FUNCTION "FC_PROG_L2" : VOID
TITLE =FC PROG OVEN LINE 2
{ S7_language := '9(1) Angielski (Stany Zjednoczone)  11.01.2022  09:45:15' }
VERSION : 0.1


VAR_TEMP
  DoorOK : BOOL ;
  ECooling_SP : REAL ;
END_VAR
BEGIN
NETWORK
TITLE =SET FULL PRODUCTION OR REDUCED PRODUCTION MODE
//THIS MODE WILL BE USE AFTER IN SETTING SETPOINTS FOR OVEN FANS (=55FAN01,
//=60FAN01)
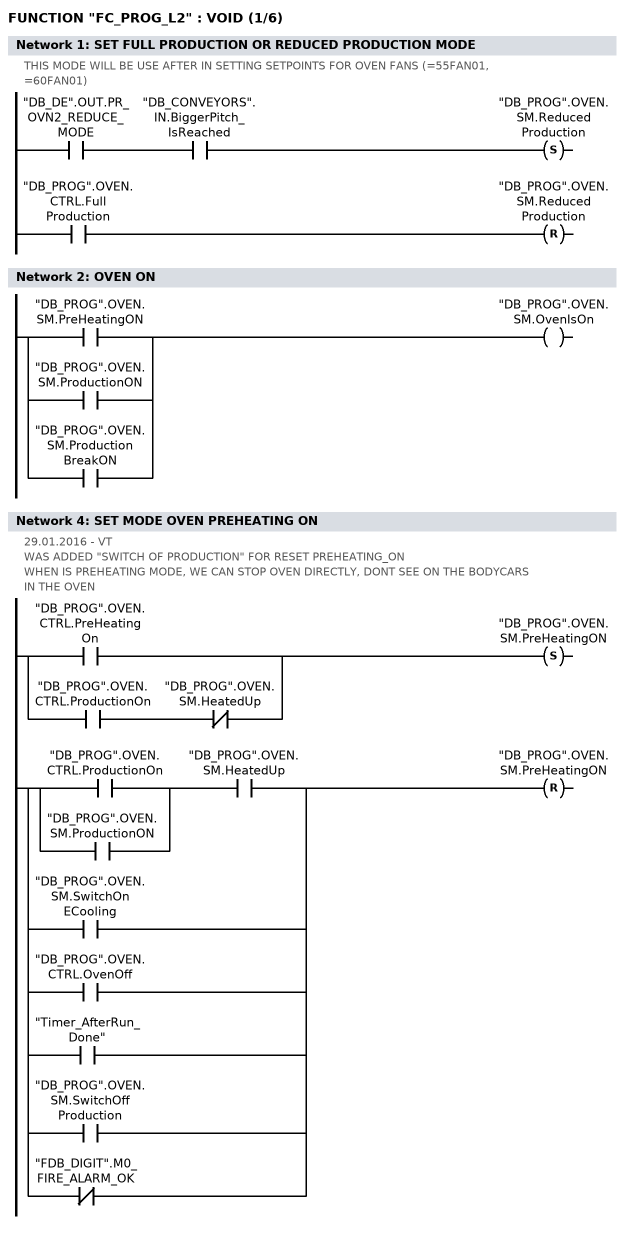
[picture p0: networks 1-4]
      U     "DB_DE".OUT.PR_OVN2_REDUCE_MODE;
      U     "DB_CONVEYORS".IN.BiggerPitch_IsReached;
      S     "DB_PROG".OVEN.SM.ReducedProduction;
      U     "DB_PROG".OVEN.CTRL.FullProduction;
      R     "DB_PROG".OVEN.SM.ReducedProduction;
      NOP   0;
NETWORK
TITLE =OVEN ON

      O     "DB_PROG".OVEN.SM.PreHeatingON;
      O     "DB_PROG".OVEN.SM.ProductionON;
      O     "DB_PROG".OVEN.SM.ProductionBreakON;
      =     "DB_PROG".OVEN.SM.OvenIsOn;
NETWORK
TITLE =SET MODE OF OVEN
//
//************************** SET MODE OF OVEN **********************************
//
NETWORK
TITLE =SET MODE OVEN PREHEATING ON
//29.01.2016 - VT
//WAS ADDED "SWITCH OF PRODUCTION" FOR RESET PREHEATING_ON
//WHEN IS PREHEATING MODE, WE CAN STOP OVEN DIRECTLY, DONT SEE ON THE BODYCARS
//IN THE OVEN
//
//
      U(    ;
      O     "DB_PROG".OVEN.CTRL.PreHeatingOn;
      O     ;
      U     "DB_PROG".OVEN.CTRL.ProductionOn;
      UN    "DB_PROG".OVEN.SM.HeatedUp;
      )     ;
      S     "DB_PROG".OVEN.SM.PreHeatingON;
      U(    ;
      U(    ;
      O     "DB_PROG".OVEN.CTRL.ProductionOn;
      O     "DB_PROG".OVEN.SM.ProductionON;
      )     ;
      U     "DB_PROG".OVEN.SM.HeatedUp;
      O     "DB_PROG".OVEN.SM.SwitchOnECooling;
      O     "DB_PROG".OVEN.CTRL.OvenOff;
      O     "Timer_AfterRun_Done";
      O     "DB_PROG".OVEN.SM.SwitchOffProduction;
      ON    "FDB_DIGIT".M0_FIRE_ALARM_OK;
      )     ;
      R     "DB_PROG".OVEN.SM.PreHeatingON;
      NOP   0;
NETWORK
TITLE =SET MODE OVEN PRODUCTION ON
//29.01.2016 - VT
//WAS ADDED ADDITIONAL LOCK FOR RESER PRODUCTION MODE -
//"OVEN_OFF_AFTER_RUN" (M410.0)
//IT MEANS, THAT WE CAN'T STOP OVEN, WHEN WITH BODYCARS INSIDE
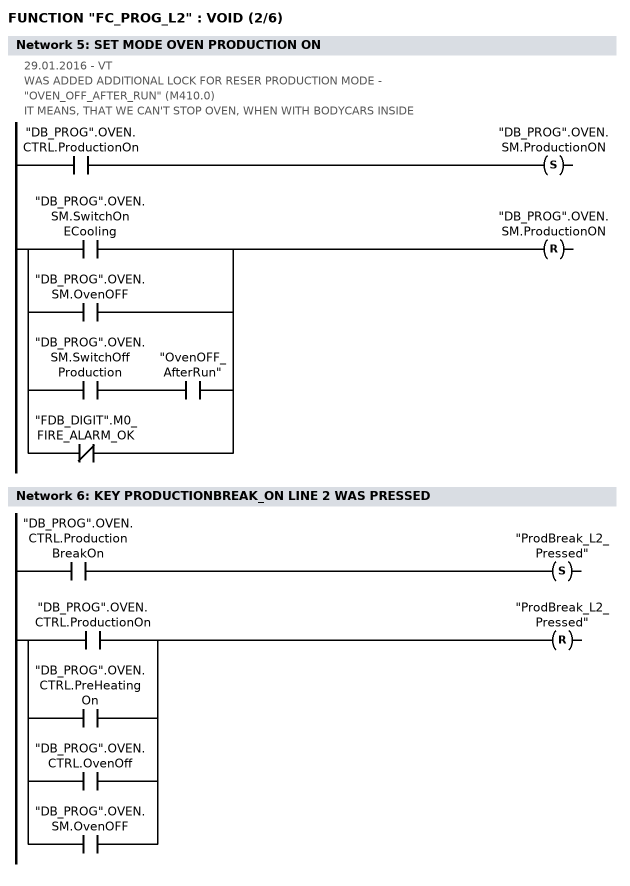
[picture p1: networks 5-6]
      U     "DB_PROG".OVEN.CTRL.ProductionOn;
      S     "DB_PROG".OVEN.SM.ProductionON;
      U(    ;
      O     "DB_PROG".OVEN.SM.SwitchOnECooling;
      O     "DB_PROG".OVEN.SM.OvenOFF;
      O     ;
      U     "DB_PROG".OVEN.SM.SwitchOffProduction;
      U     "OvenOFF_AfterRun";
      ON    "FDB_DIGIT".M0_FIRE_ALARM_OK;
      )     ;
      R     "DB_PROG".OVEN.SM.ProductionON;
      NOP   0;
NETWORK
TITLE =KEY PRODUCTIONBREAK_ON LINE 2 WAS PRESSED

      U     "DB_PROG".OVEN.CTRL.ProductionBreakOn;
      S     "ProdBreak_L2_Pressed";
      U(    ;
      O     "DB_PROG".OVEN.CTRL.ProductionOn;
      O     "DB_PROG".OVEN.CTRL.PreHeatingOn;
      O     "DB_PROG".OVEN.CTRL.OvenOff;
      O     "DB_PROG".OVEN.SM.OvenOFF;
      )     ;
      R     "ProdBreak_L2_Pressed";
      NOP   0;
NETWORK
TITLE =SET MODE OVEN PRODUCTION BREAK ON
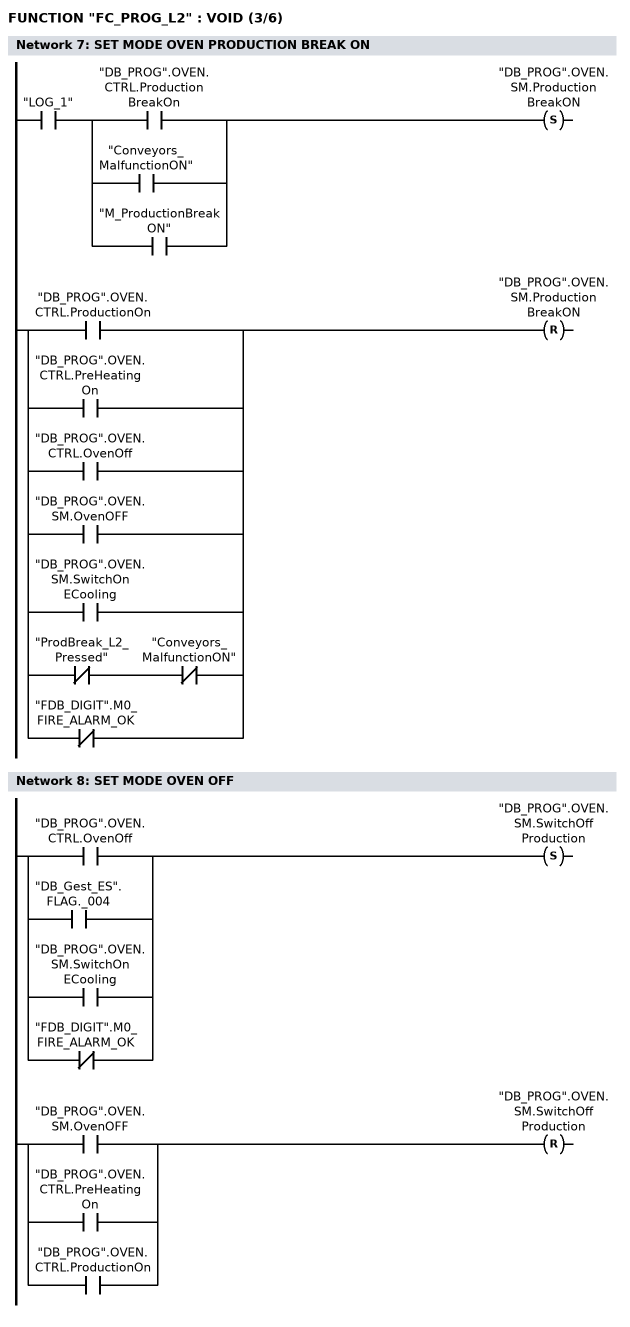
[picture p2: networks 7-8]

      U     "LOG_1";
      U(    ;
      O     "DB_PROG".OVEN.CTRL.ProductionBreakOn;
      O     "Conveyors_MalfunctionON";
      O     "M_ProductionBreakON";
      )     ;
      S     "DB_PROG".OVEN.SM.ProductionBreakON;
      U(    ;
      O     "DB_PROG".OVEN.CTRL.ProductionOn;
      O     "DB_PROG".OVEN.CTRL.PreHeatingOn;
      O     "DB_PROG".OVEN.CTRL.OvenOff;
      O     "DB_PROG".OVEN.SM.OvenOFF;
      O     "DB_PROG".OVEN.SM.SwitchOnECooling;
      O     ;
      UN    "ProdBreak_L2_Pressed";
      UN    "Conveyors_MalfunctionON";
      ON    "FDB_DIGIT".M0_FIRE_ALARM_OK;
      )     ;
      R     "DB_PROG".OVEN.SM.ProductionBreakON;
      NOP   0;
NETWORK
TITLE =SET MODE OVEN OFF

      U(    ;
      O     "DB_PROG".OVEN.CTRL.OvenOff;
      O     "DB_Gest_ES".FLAG._004;
      O     "DB_PROG".OVEN.SM.SwitchOnECooling;
      ON    "FDB_DIGIT".M0_FIRE_ALARM_OK;
      )     ;
      S     "DB_PROG".OVEN.SM.SwitchOffProduction;
      U(    ;
      O     "DB_PROG".OVEN.SM.OvenOFF;
      O     "DB_PROG".OVEN.CTRL.PreHeatingOn;
      O     "DB_PROG".OVEN.CTRL.ProductionOn;
      )     ;
      R     "DB_PROG".OVEN.SM.SwitchOffProduction;
      NOP   0;
NETWORK
TITLE =AFTER VENTILATION IS FINISHED, OVEN IS OFF
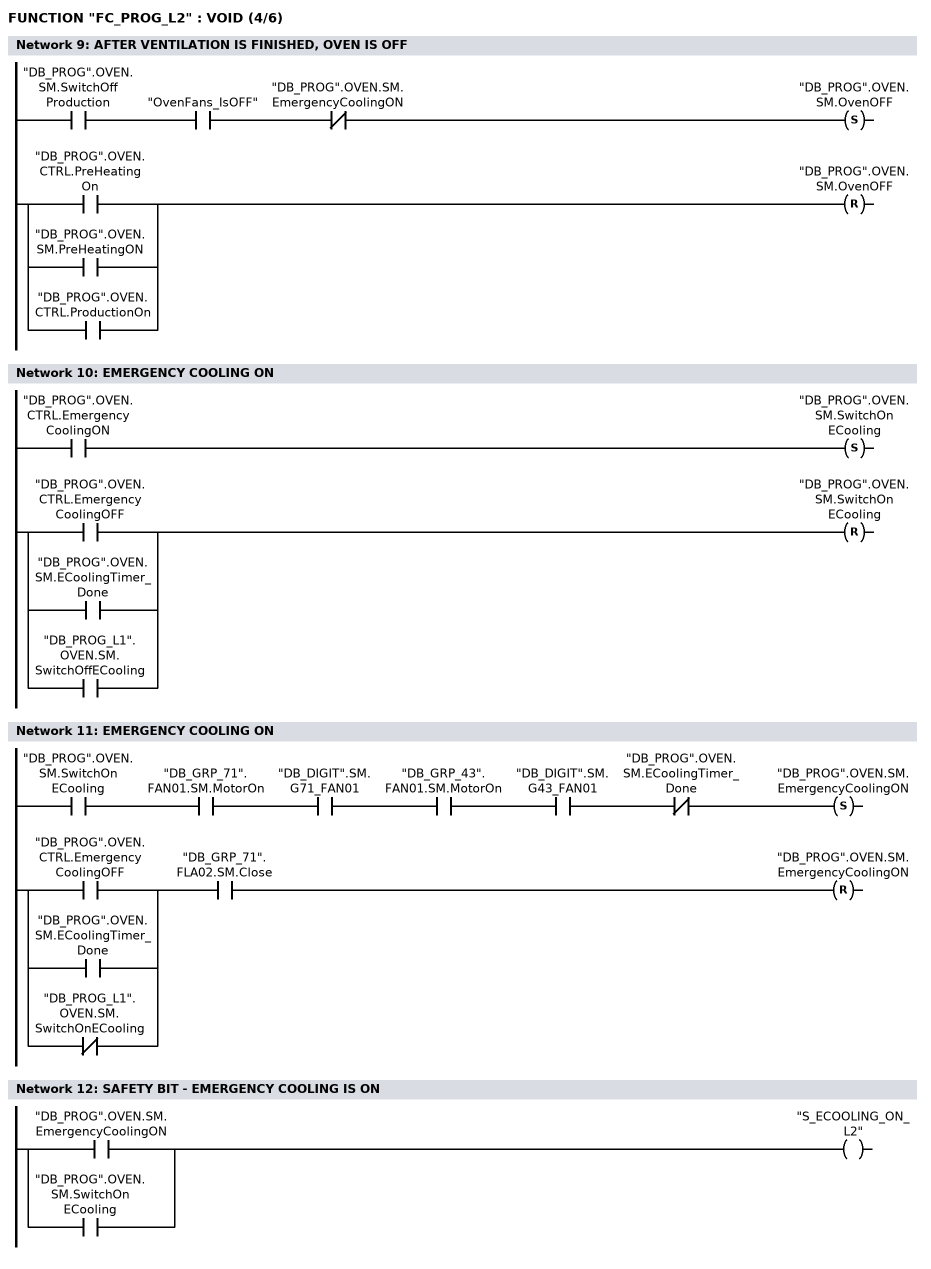
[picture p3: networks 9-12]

      U     "DB_PROG".OVEN.SM.SwitchOffProduction;
      U     "OvenFans_IsOFF";
      UN    "DB_PROG".OVEN.SM.EmergencyCoolingON;
      S     "DB_PROG".OVEN.SM.OvenOFF;
      U(    ;
      O     "DB_PROG".OVEN.CTRL.PreHeatingOn;
      O     "DB_PROG".OVEN.SM.PreHeatingON;
      O     "DB_PROG".OVEN.CTRL.ProductionOn;
      )     ;
      R     "DB_PROG".OVEN.SM.OvenOFF;
      NOP   0;
NETWORK
TITLE =EMERGENCY COOLING ON

      U     "DB_PROG".OVEN.CTRL.EmergencyCoolingON;
      S     "DB_PROG".OVEN.SM.SwitchOnECooling;
      U(    ;
      O     "DB_PROG".OVEN.CTRL.EmergencyCoolingOFF;
      O     "DB_PROG".OVEN.SM.ECoolingTimer_Done;
      O     "DB_PROG_L1".OVEN.SM.SwitchOffECooling;
      )     ;
      R     "DB_PROG".OVEN.SM.SwitchOnECooling;
      NOP   0;
NETWORK
TITLE =EMERGENCY COOLING ON

      U     "DB_PROG".OVEN.SM.SwitchOnECooling;
      U     "DB_GRP_71".FAN01.SM.MotorOn;
      U     "DB_DIGIT".SM.G71_FAN01;
      U     "DB_GRP_43".FAN01.SM.MotorOn;
      U     "DB_DIGIT".SM.G43_FAN01;
      UN    "DB_PROG".OVEN.SM.ECoolingTimer_Done;
      S     "DB_PROG".OVEN.SM.EmergencyCoolingON;
      U(    ;
      O     "DB_PROG".OVEN.CTRL.EmergencyCoolingOFF;
      O     "DB_PROG".OVEN.SM.ECoolingTimer_Done;
      ON    "DB_PROG_L1".OVEN.SM.SwitchOnECooling;
      )     ;
      U     "DB_GRP_71".FLA02.SM.Close;
      R     "DB_PROG".OVEN.SM.EmergencyCoolingON;
      NOP   0;
NETWORK
TITLE =SAFETY BIT - EMERGENCY COOLING IS ON

      O     "DB_PROG".OVEN.SM.EmergencyCoolingON;
      O     "DB_PROG".OVEN.SM.SwitchOnECooling;
      =     "S_ECOOLING_ON_L2";
NETWORK
TITLE =SWITCHING EMERGENCY COOLING OFF
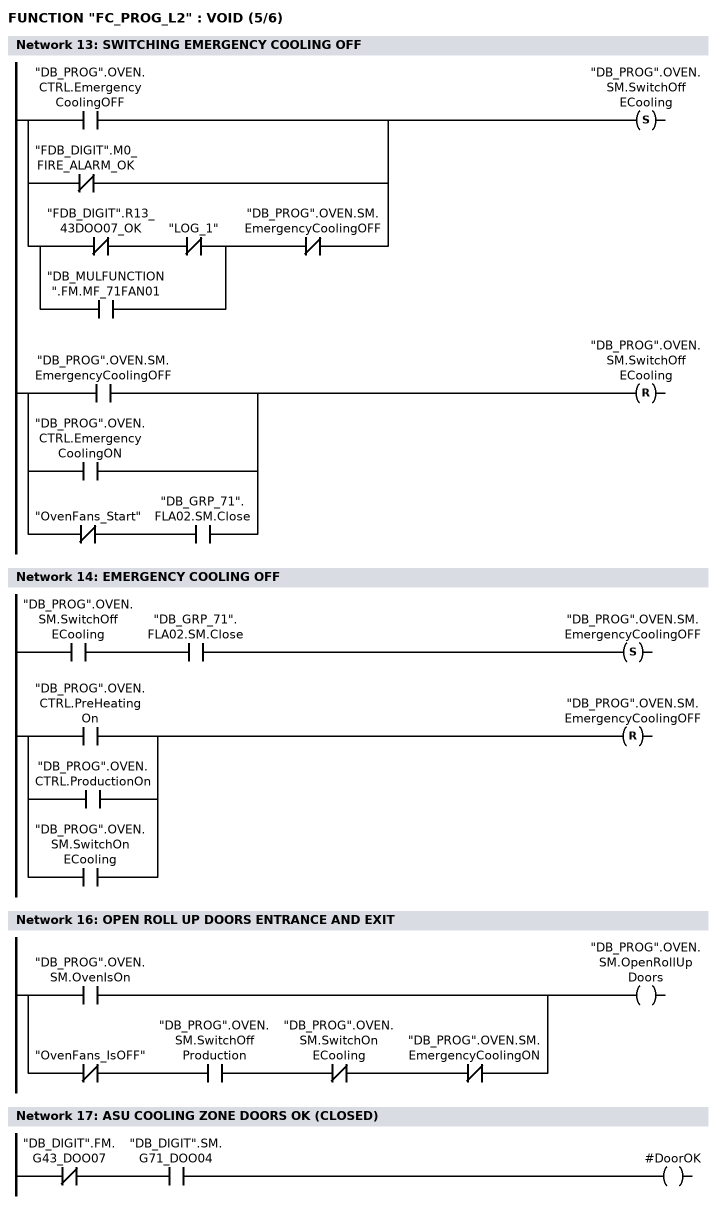
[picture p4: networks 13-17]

      U(    ;
      O     "DB_PROG".OVEN.CTRL.EmergencyCoolingOFF;
      ON    "FDB_DIGIT".M0_FIRE_ALARM_OK;
      O     ;
      U(    ;
      UN    "FDB_DIGIT".R13_43DOO07_OK;
      UN    "LOG_1";
      O     "DB_MULFUNCTION".FM.MF_71FAN01;
      )     ;
      UN    "DB_PROG".OVEN.SM.EmergencyCoolingOFF;
      )     ;
      S     "DB_PROG".OVEN.SM.SwitchOffECooling;
      U(    ;
      O     "DB_PROG".OVEN.SM.EmergencyCoolingOFF;
      O     "DB_PROG".OVEN.CTRL.EmergencyCoolingON;
      O     ;
      UN    "OvenFans_Start";
      U     "DB_GRP_71".FLA02.SM.Close;
      )     ;
      R     "DB_PROG".OVEN.SM.SwitchOffECooling;
      NOP   0;
NETWORK
TITLE =EMERGENCY COOLING OFF

      U     "DB_PROG".OVEN.SM.SwitchOffECooling;
      U     "DB_GRP_71".FLA02.SM.Close;
      S     "DB_PROG".OVEN.SM.EmergencyCoolingOFF;
      U(    ;
      O     "DB_PROG".OVEN.CTRL.PreHeatingOn;
      O     "DB_PROG".OVEN.CTRL.ProductionOn;
      O     "DB_PROG".OVEN.SM.SwitchOnECooling;
      )     ;
      R     "DB_PROG".OVEN.SM.EmergencyCoolingOFF;
      NOP   0;
NETWORK
TITLE =PRE-HEATING MODE
//
//**************************** SET OVEN PRE-HEATING MODE ************************
//
NETWORK
TITLE =OPEN ROLL UP DOORS ENTRANCE AND EXIT

      O     "DB_PROG".OVEN.SM.OvenIsOn;
      O     ;
      UN    "OvenFans_IsOFF";
      U     "DB_PROG".OVEN.SM.SwitchOffProduction;
      UN    "DB_PROG".OVEN.SM.SwitchOnECooling;
      UN    "DB_PROG".OVEN.SM.EmergencyCoolingON;
      =     "DB_PROG".OVEN.SM.OpenRollUpDoors;
NETWORK
TITLE =ASU COOLING ZONE DOORS OK (CLOSED)

      UN    "DB_DIGIT".FM.G43_DOO07;
      U     "DB_DIGIT".SM.G71_DOO04;
      =     #DoorOK;
NETWORK
TITLE =OVEN CHAIN ON
//FROM E-MAIL FROM EN DON'T LOOK ON THE SIGNAL FROM
//CONVEYORS
//"DoorExit_IsMovedFree" - STOP CHAIN IMMEDIATELY AFTER GIVE BACK
//"DoorEntrance_IsMovedFree" AND IS EMERGENCY COOLING ON.
//
//23.04.2016 - VT
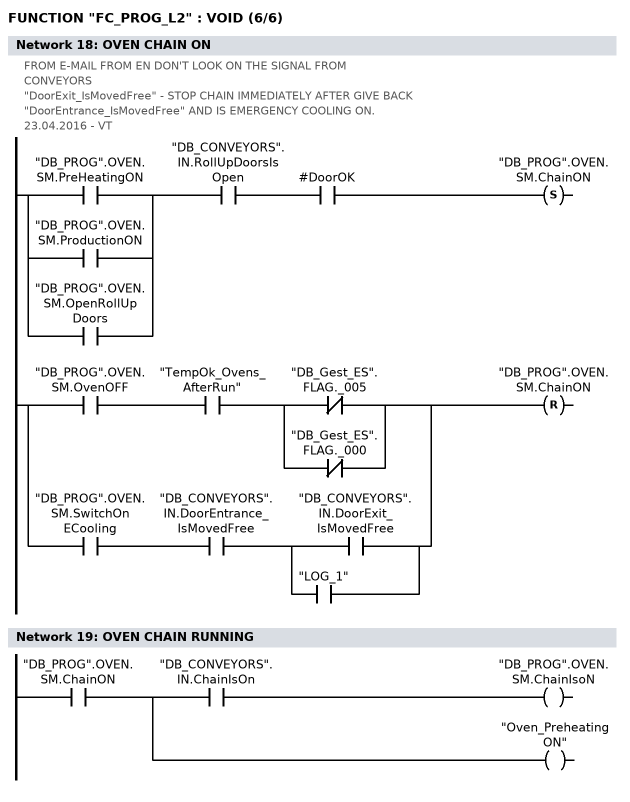
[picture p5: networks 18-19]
      U(    ;
      O     "DB_PROG".OVEN.SM.PreHeatingON;
      O     "DB_PROG".OVEN.SM.ProductionON;
      O     "DB_PROG".OVEN.SM.OpenRollUpDoors;
      )     ;
      U     "DB_CONVEYORS".IN.RollUpDoorsIsOpen;
      U     #DoorOK;
      S     "DB_PROG".OVEN.SM.ChainON;
      U(    ;
      U     "DB_PROG".OVEN.SM.OvenOFF;
      U     "TempOk_Ovens_AfterRun";
      U(    ;
      ON    "DB_Gest_ES".FLAG._005;
      ON    "DB_Gest_ES".FLAG._000;
      )     ;
      O     ;
      U     "DB_PROG".OVEN.SM.SwitchOnECooling;
      U     "DB_CONVEYORS".IN.DoorEntrance_IsMovedFree;
      U(    ;
      O     "DB_CONVEYORS".IN.DoorExit_IsMovedFree;
      O     "LOG_1";
      )     ;
      )     ;
      R     "DB_PROG".OVEN.SM.ChainON;
      NOP   0;
NETWORK
TITLE =OVEN CHAIN RUNNING

      U     "DB_PROG".OVEN.SM.ChainON;
      =     L      6.0;
      U     L      6.0;
      U     "DB_CONVEYORS".IN.ChainIsOn;
      =     "DB_PROG".OVEN.SM.ChainIsoN;
      U     L      6.0;
      BLD   102;
      =     "Oven_PreheatingON";
NETWORK
TITLE =CLOSE FLAPS =43/=44/=51/=52/=61FLA02 AND OPEN FLAPS =55FLA02/06

      U(    ;
      U     "DB_PROG".OVEN.SM.PreHeatingON;
      S     "CloseFlap_ToMainPosition";
      U     "DB_PROG".OVEN.SM.MainPosition;
      R     "CloseFlap_ToMainPosition";
      U     "CloseFlap_ToMainPosition";
      )     ;
      S     "Open_55FLA06";
      U(    ;
      UN    "DB_PROG".OVEN.SM.OvenIsOn;
      U     "DB_GRP_60".FAN01.SM.MotorOff;
      U     "DB_GRP_55".FAN01.SM.MotorOff;
      L     S5T#30S;
      SE    "T_5_0_1";
      NOP   0;
      NOP   0;
      NOP   0;
      U     "T_5_0_1";
      )     ;
      R     "Open_55FLA06";
      NOP   0;
NETWORK
TITLE =CHECK LIMIT SWITCHES OF =43/=44/=51/=52FLA02
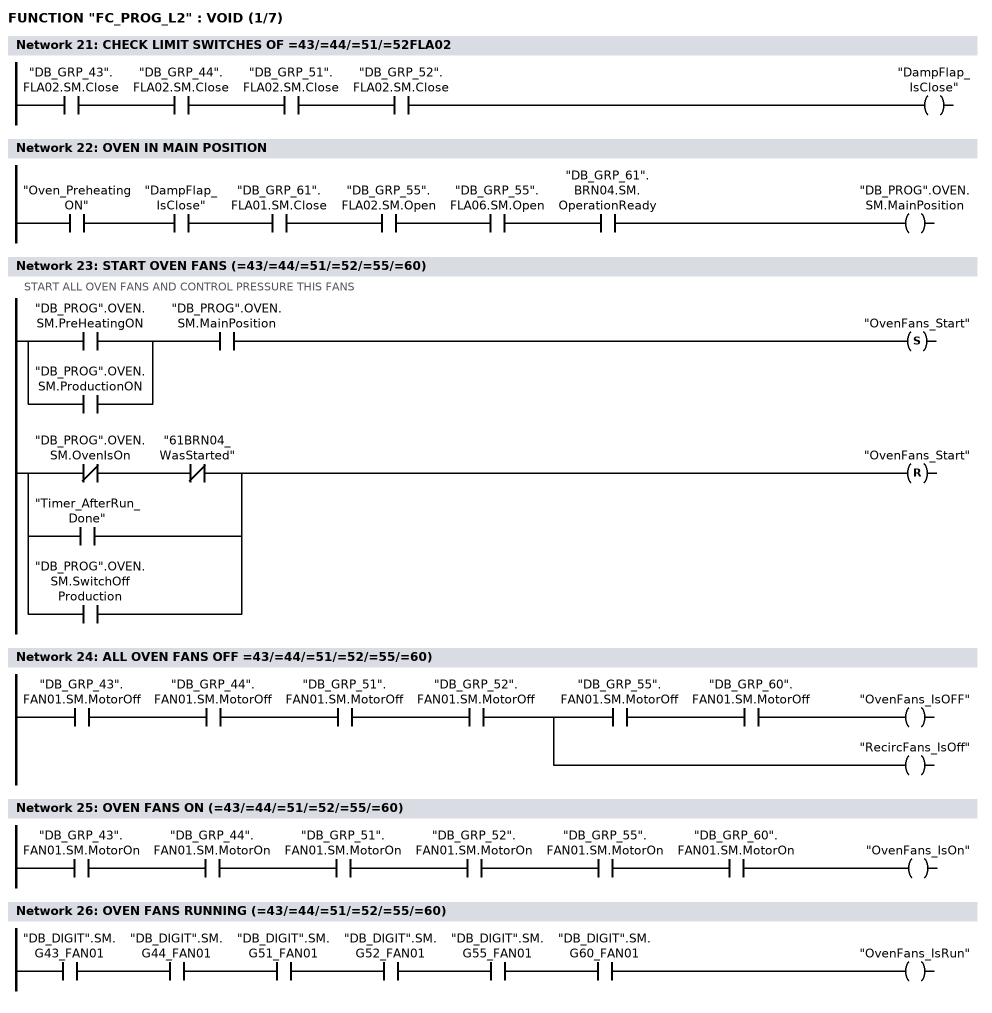
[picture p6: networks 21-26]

      U     "DB_GRP_43".FLA02.SM.Close;
      U     "DB_GRP_44".FLA02.SM.Close;
      U     "DB_GRP_51".FLA02.SM.Close;
      U     "DB_GRP_52".FLA02.SM.Close;
      =     "DampFlap_IsClose";
NETWORK
TITLE =OVEN IN MAIN POSITION

      U     "Oven_PreheatingON";
      U     "DampFlap_IsClose";
      U     "DB_GRP_61".FLA01.SM.Close;
      U     "DB_GRP_55".FLA02.SM.Open;
      U     "DB_GRP_55".FLA06.SM.Open;
      U     "DB_GRP_61".BRN04.SM.OperationReady;
      =     "DB_PROG".OVEN.SM.MainPosition;
NETWORK
TITLE =START OVEN FANS (=43/=44/=51/=52/=55/=60)
//START ALL OVEN FANS AND CONTROL PRESSURE THIS FANS
      U(    ;
      O     "DB_PROG".OVEN.SM.PreHeatingON;
      O     "DB_PROG".OVEN.SM.ProductionON;
      )     ;
      U     "DB_PROG".OVEN.SM.MainPosition;
      S     "OvenFans_Start";
      U(    ;
      UN    "DB_PROG".OVEN.SM.OvenIsOn;
      UN    "61BRN04_WasStarted";
      O     "Timer_AfterRun_Done";
      O     "DB_PROG".OVEN.SM.SwitchOffProduction;
      )     ;
      R     "OvenFans_Start";
      NOP   0;
NETWORK
TITLE =ALL OVEN FANS OFF =43/=44/=51/=52/=55/=60)

      U     "DB_GRP_43".FAN01.SM.MotorOff;
      U     "DB_GRP_44".FAN01.SM.MotorOff;
      U     "DB_GRP_51".FAN01.SM.MotorOff;
      U     "DB_GRP_52".FAN01.SM.MotorOff;
      =     L      6.0;
      U     L      6.0;
      U     "DB_GRP_55".FAN01.SM.MotorOff;
      U     "DB_GRP_60".FAN01.SM.MotorOff;
      =     "OvenFans_IsOFF";
      U     L      6.0;
      BLD   102;
      =     "RecircFans_IsOff";
NETWORK
TITLE =OVEN FANS ON (=43/=44/=51/=52/=55/=60)

      U     "DB_GRP_43".FAN01.SM.MotorOn;
      U     "DB_GRP_44".FAN01.SM.MotorOn;
      U     "DB_GRP_51".FAN01.SM.MotorOn;
      U     "DB_GRP_52".FAN01.SM.MotorOn;
      U     "DB_GRP_55".FAN01.SM.MotorOn;
      U     "DB_GRP_60".FAN01.SM.MotorOn;
      =     "OvenFans_IsOn";
NETWORK
TITLE =OVEN FANS RUNNING (=43/=44/=51/=52/=55/=60)

      U     "DB_DIGIT".SM.G43_FAN01;
      U     "DB_DIGIT".SM.G44_FAN01;
      U     "DB_DIGIT".SM.G51_FAN01;
      U     "DB_DIGIT".SM.G52_FAN01;
      U     "DB_DIGIT".SM.G55_FAN01;
      U     "DB_DIGIT".SM.G60_FAN01;
      =     "OvenFans_IsRun";
NETWORK
TITLE =PRE-PURGING TIMER
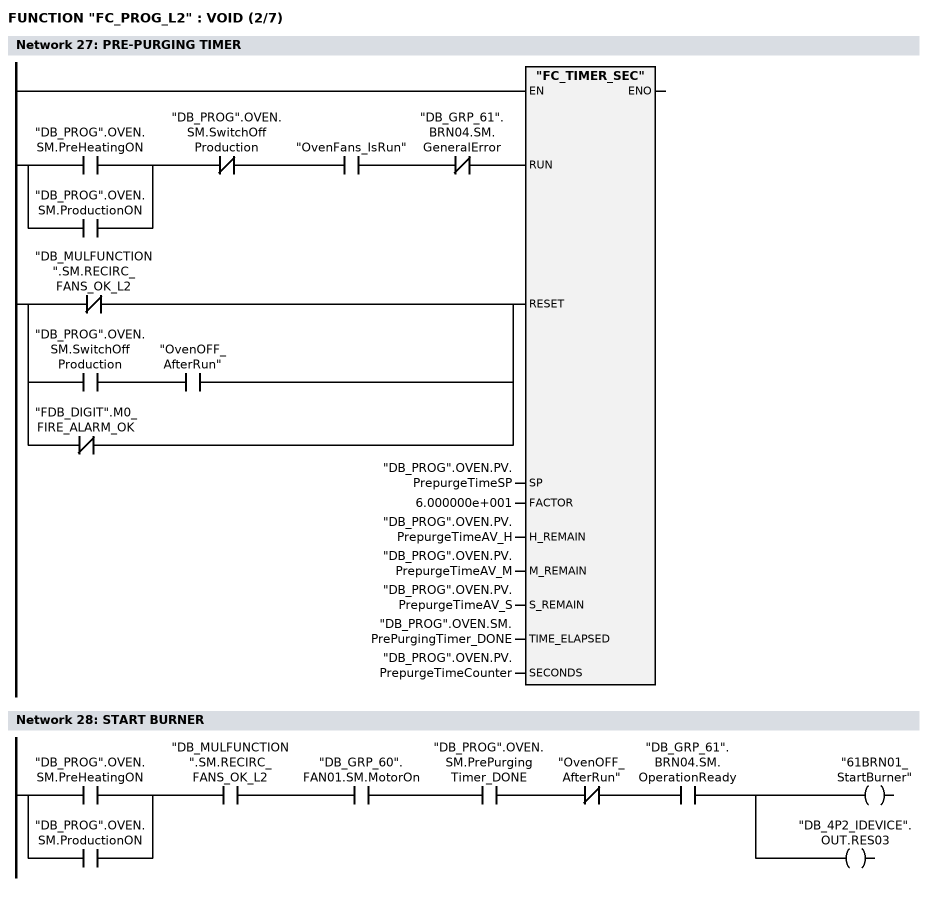
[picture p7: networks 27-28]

      U(    ;
      O     "DB_PROG".OVEN.SM.PreHeatingON;
      O     "DB_PROG".OVEN.SM.ProductionON;
      )     ;
      UN    "DB_PROG".OVEN.SM.SwitchOffProduction;
      U     "OvenFans_IsRun";
      UN    "DB_GRP_61".BRN04.SM.GeneralError;
      =     L      6.0;
      BLD   103;
      U(    ;
      ON    "DB_MULFUNCTION".SM.RECIRC_FANS_OK_L2;
      O     ;
      U     "DB_PROG".OVEN.SM.SwitchOffProduction;
      U     "OvenOFF_AfterRun";
      ON    "FDB_DIGIT".M0_FIRE_ALARM_OK;
      )     ;
      =     L      6.1;
      BLD   103;
      CALL "FC_TIMER_SEC" (
           RUN                      := L      6.0,
           RESET                    := L      6.1,
           SP                       := "DB_PROG".OVEN.PV.PrepurgeTimeSP,
           FACTOR                   := 6.000000e+001,
           H_REMAIN                 := "DB_PROG".OVEN.PV.PrepurgeTimeAV_H,
           M_REMAIN                 := "DB_PROG".OVEN.PV.PrepurgeTimeAV_M,
           S_REMAIN                 := "DB_PROG".OVEN.PV.PrepurgeTimeAV_S,
           TIME_ELAPSED             := "DB_PROG".OVEN.SM.PrePurgingTimer_DONE,
           SECONDS                  := "DB_PROG".OVEN.PV.PrepurgeTimeCounter);
      NOP   0;
NETWORK
TITLE =START BURNER

      U(    ;
      O     "DB_PROG".OVEN.SM.PreHeatingON;
      O     "DB_PROG".OVEN.SM.ProductionON;
      )     ;
      U     "DB_MULFUNCTION".SM.RECIRC_FANS_OK_L2;
      U     "DB_GRP_60".FAN01.SM.MotorOn;
      U     "DB_PROG".OVEN.SM.PrePurgingTimer_DONE;
      UN    "OvenOFF_AfterRun";
      U     "DB_GRP_61".BRN04.SM.OperationReady;
      =     "61BRN01_StartBurner";
      =     "DB_4P2_IDEVICE".OUT.RES03;
NETWORK
TITLE =OVEN GROUP =43/=44/=51/=52/=55 TEMPERATURE OK
//
//"DB_GRP_44".CLT03.PV.Limit_03
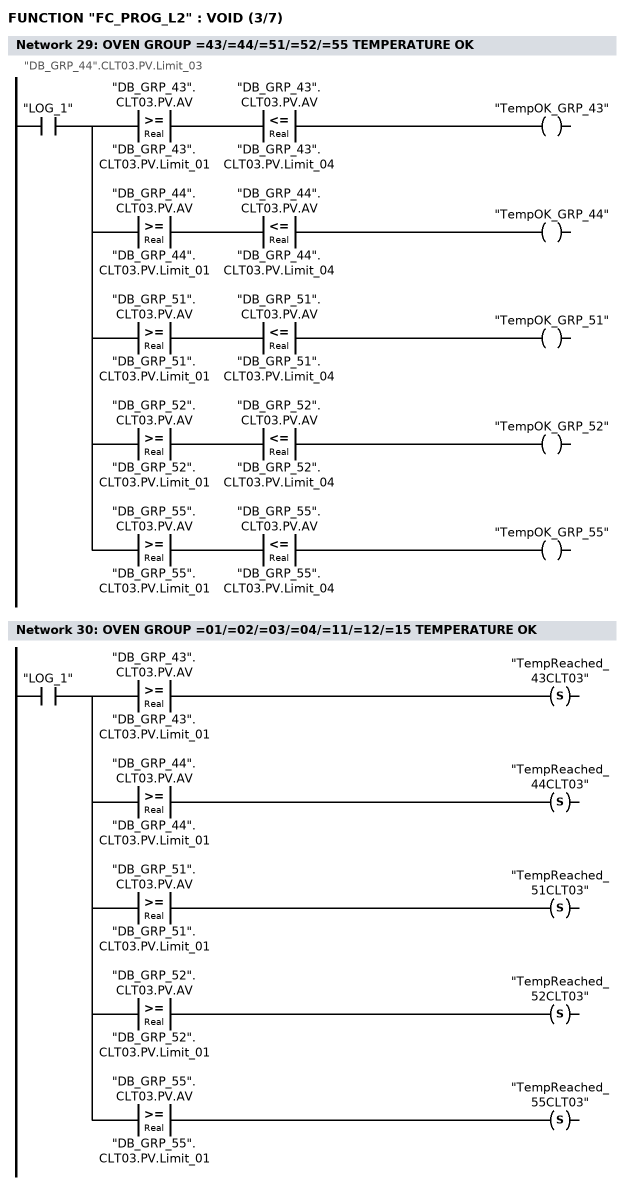
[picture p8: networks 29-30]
      U     "LOG_1";
      =     L      6.0;
      U     L      6.0;
      U(    ;
      L     "DB_GRP_43".CLT03.PV.AV;
      L     "DB_GRP_43".CLT03.PV.Limit_01;
      >=R   ;
      )     ;
      U(    ;
      L     "DB_GRP_43".CLT03.PV.AV;
      L     "DB_GRP_43".CLT03.PV.Limit_04;
      <=R   ;
      )     ;
      =     "TempOK_GRP_43";
      U     L      6.0;
      U(    ;
      L     "DB_GRP_44".CLT03.PV.AV;
      L     "DB_GRP_44".CLT03.PV.Limit_01;
      >=R   ;
      )     ;
      U(    ;
      L     "DB_GRP_44".CLT03.PV.AV;
      L     "DB_GRP_44".CLT03.PV.Limit_04;
      <=R   ;
      )     ;
      =     "TempOK_GRP_44";
      U     L      6.0;
      U(    ;
      L     "DB_GRP_51".CLT03.PV.AV;
      L     "DB_GRP_51".CLT03.PV.Limit_01;
      >=R   ;
      )     ;
      U(    ;
      L     "DB_GRP_51".CLT03.PV.AV;
      L     "DB_GRP_51".CLT03.PV.Limit_04;
      <=R   ;
      )     ;
      =     "TempOK_GRP_51";
      U     L      6.0;
      U(    ;
      L     "DB_GRP_52".CLT03.PV.AV;
      L     "DB_GRP_52".CLT03.PV.Limit_01;
      >=R   ;
      )     ;
      U(    ;
      L     "DB_GRP_52".CLT03.PV.AV;
      L     "DB_GRP_52".CLT03.PV.Limit_04;
      <=R   ;
      )     ;
      =     "TempOK_GRP_52";
      U     L      6.0;
      U(    ;
      L     "DB_GRP_55".CLT03.PV.AV;
      L     "DB_GRP_55".CLT03.PV.Limit_01;
      >=R   ;
      )     ;
      U(    ;
      L     "DB_GRP_55".CLT03.PV.AV;
      L     "DB_GRP_55".CLT03.PV.Limit_04;
      <=R   ;
      )     ;
      =     "TempOK_GRP_55";
NETWORK
TITLE =OVEN GROUP =01/=02/=03/=04/=11/=12/=15 TEMPERATURE OK

      U     "LOG_1";
      =     L      6.0;
      U     L      6.0;
      U(    ;
      L     "DB_GRP_43".CLT03.PV.AV;
      L     "DB_GRP_43".CLT03.PV.Limit_01;
      >=R   ;
      )     ;
      S     "TempReached_43CLT03";
      U     L      6.0;
      U(    ;
      L     "DB_GRP_44".CLT03.PV.AV;
      L     "DB_GRP_44".CLT03.PV.Limit_01;
      >=R   ;
      )     ;
      S     "TempReached_44CLT03";
      U     L      6.0;
      U(    ;
      L     "DB_GRP_51".CLT03.PV.AV;
      L     "DB_GRP_51".CLT03.PV.Limit_01;
      >=R   ;
      )     ;
      S     "TempReached_51CLT03";
      U     L      6.0;
      U(    ;
      L     "DB_GRP_52".CLT03.PV.AV;
      L     "DB_GRP_52".CLT03.PV.Limit_01;
      >=R   ;
      )     ;
      S     "TempReached_52CLT03";
      U     L      6.0;
      U(    ;
      L     "DB_GRP_55".CLT03.PV.AV;
      L     "DB_GRP_55".CLT03.PV.Limit_01;
      >=R   ;
      )     ;
      S     "TempReached_55CLT03";
NETWORK
TITLE =TEMPERATURE OK
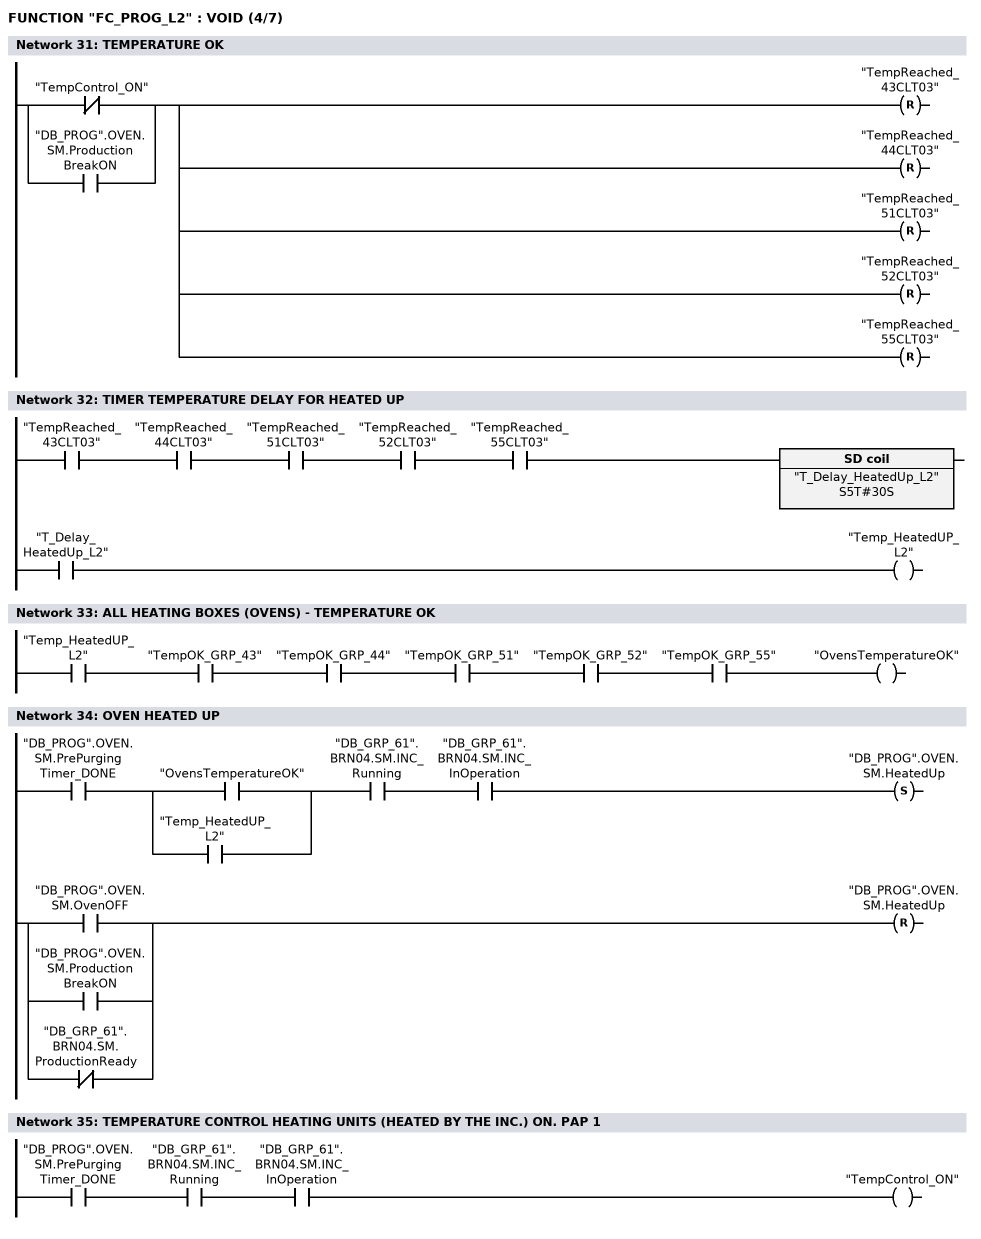
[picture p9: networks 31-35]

      ON    "TempControl_ON";
      O     "DB_PROG".OVEN.SM.ProductionBreakON;
      R     "TempReached_43CLT03";
      R     "TempReached_44CLT03";
      R     "TempReached_51CLT03";
      R     "TempReached_52CLT03";
      R     "TempReached_55CLT03";
NETWORK
TITLE =TIMER TEMPERATURE DELAY FOR HEATED UP

      U     "TempReached_43CLT03";
      U     "TempReached_44CLT03";
      U     "TempReached_51CLT03";
      U     "TempReached_52CLT03";
      U     "TempReached_55CLT03";
      L     S5T#30S;
      SE    "T_Delay_HeatedUp_L2";
      NOP   0;
      NOP   0;
      NOP   0;
      U     "T_Delay_HeatedUp_L2";
      =     "Temp_HeatedUP_L2";
NETWORK
TITLE =ALL HEATING BOXES (OVENS) - TEMPERATURE OK

      U     "Temp_HeatedUP_L2";
      U     "TempOK_GRP_43";
      U     "TempOK_GRP_44";
      U     "TempOK_GRP_51";
      U     "TempOK_GRP_52";
      U     "TempOK_GRP_55";
      =     "OvensTemperatureOK";
NETWORK
TITLE =OVEN HEATED UP

      U     "DB_PROG".OVEN.SM.PrePurgingTimer_DONE;
      U(    ;
      O     "OvensTemperatureOK";
      O     "Temp_HeatedUP_L2";
      )     ;
      U     "DB_GRP_61".BRN04.SM.INC_Running;
      U     "DB_GRP_61".BRN04.SM.INC_InOperation;
      S     "DB_PROG".OVEN.SM.HeatedUp;
      U(    ;
      O     "DB_PROG".OVEN.SM.OvenOFF;
      O     "DB_PROG".OVEN.SM.ProductionBreakON;
      ON    "DB_GRP_61".BRN04.SM.ProductionReady;
      )     ;
      R     "DB_PROG".OVEN.SM.HeatedUp;
      NOP   0;
NETWORK
TITLE =TEMPERATURE CONTROL HEATING UNITS (HEATED BY THE INC.) ON. PAP 1

      U     "DB_PROG".OVEN.SM.PrePurgingTimer_DONE;
      U     "DB_GRP_61".BRN04.SM.INC_Running;
      U     "DB_GRP_61".BRN04.SM.INC_InOperation;
      =     "TempControl_ON";
NETWORK
TITLE =BARNER =61BRN04 WAS STARTED
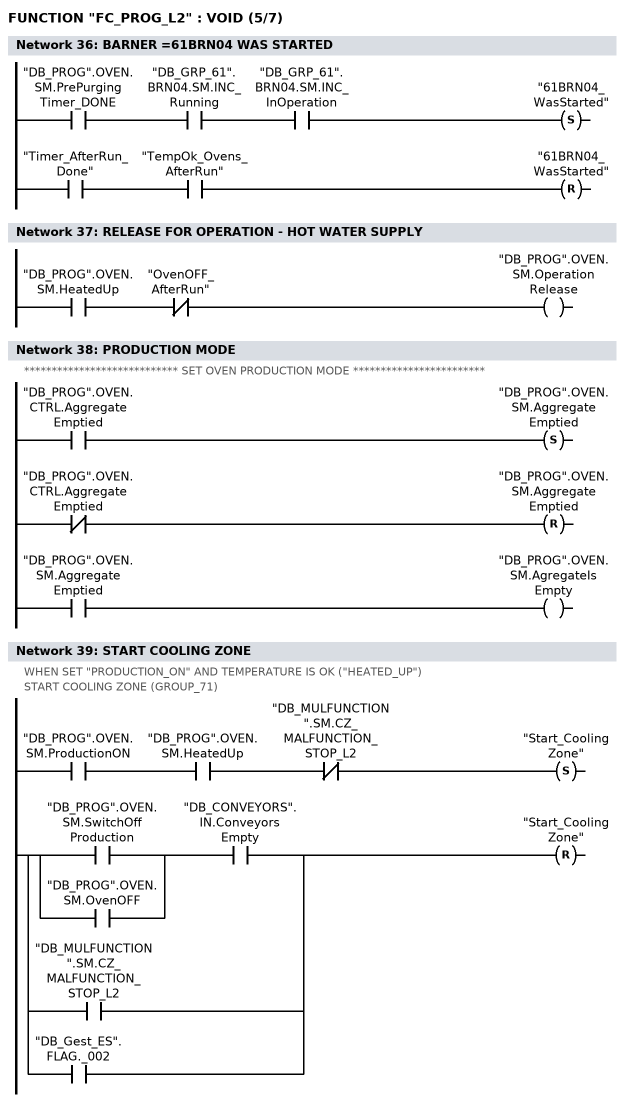
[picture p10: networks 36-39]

      U     "DB_PROG".OVEN.SM.PrePurgingTimer_DONE;
      U     "DB_GRP_61".BRN04.SM.INC_Running;
      U     "DB_GRP_61".BRN04.SM.INC_InOperation;
      S     "61BRN04_WasStarted";
      U     "Timer_AfterRun_Done";
      U     "TempOk_Ovens_AfterRun";
      R     "61BRN04_WasStarted";
      NOP   0;
NETWORK
TITLE =RELEASE FOR OPERATION - HOT WATER SUPPLY

      U     "DB_PROG".OVEN.SM.HeatedUp;
      UN    "OvenOFF_AfterRun";
      =     "DB_PROG".OVEN.SM.OperationRelease;
NETWORK
TITLE =PRODUCTION MODE
//
//**************************** SET OVEN PRODUCTION MODE ************************
//
      U     "DB_PROG".OVEN.CTRL.AggregateEmptied;
      S     "DB_PROG".OVEN.SM.AggregateEmptied;
      UN    "DB_PROG".OVEN.CTRL.AggregateEmptied;
      R     "DB_PROG".OVEN.SM.AggregateEmptied;
      U     "DB_PROG".OVEN.SM.AggregateEmptied;
      =     "DB_PROG".OVEN.SM.AgregateIsEmpty;
NETWORK
TITLE =START COOLING ZONE
//WHEN SET "PRODUCTION_ON" AND TEMPERATURE IS OK ("HEATED_UP")
//START COOLING ZONE (GROUP_71)
      U     "DB_PROG".OVEN.SM.ProductionON;
      U     "DB_PROG".OVEN.SM.HeatedUp;
      UN    "DB_MULFUNCTION".SM.CZ_MALFUNCTION_STOP_L2;
      S     "Start_CoolingZone";
      U(    ;
      U(    ;
      O     "DB_PROG".OVEN.SM.SwitchOffProduction;
      O     "DB_PROG".OVEN.SM.OvenOFF;
      )     ;
      U     "DB_CONVEYORS".IN.ConveyorsEmpty;
      O     "DB_MULFUNCTION".SM.CZ_MALFUNCTION_STOP_L2;
      O     "DB_Gest_ES".FLAG._002;
      )     ;
      R     "Start_CoolingZone";
      NOP   0;
NETWORK
TITLE =COOLING ZONE - MOVE FLAPS TO MAIN POSITION
//MOVE FLAPS TO MAIN POSITION
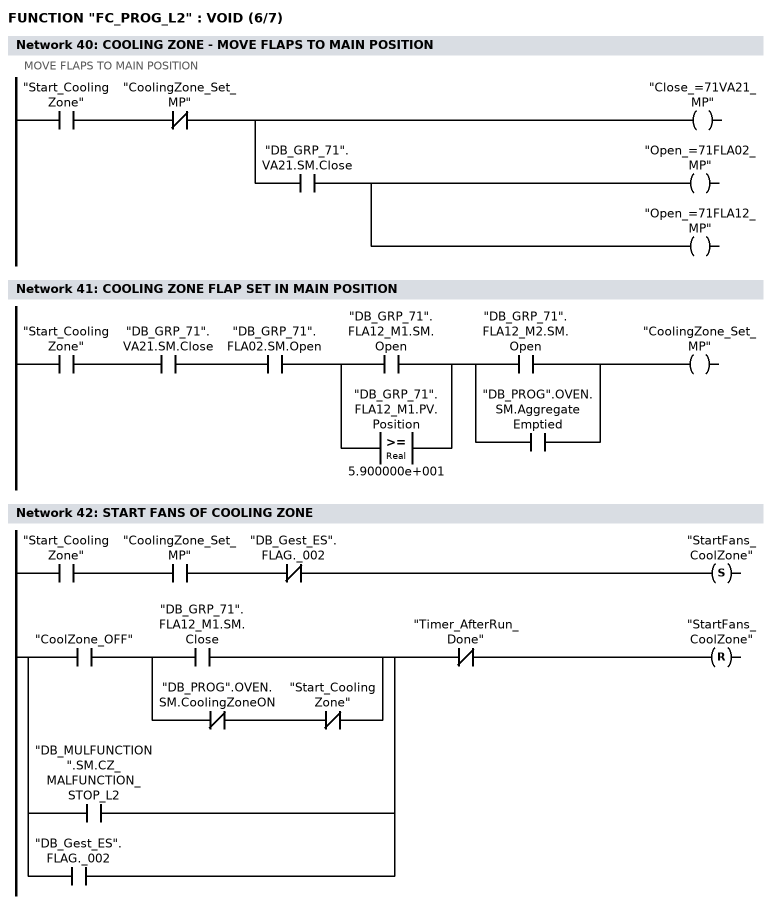
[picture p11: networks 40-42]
      U     "Start_CoolingZone";
      UN    "CoolingZone_Set_MP";
      =     L      6.0;
      U     L      6.0;
      BLD   102;
      =     "Close_=71VA21_MP";
      U     L      6.0;
      U     "DB_GRP_71".VA21.SM.Close;
      =     "Open_=71FLA02_MP";
      =     "Open_=71FLA12_MP";
NETWORK
TITLE =COOLING ZONE FLAP SET IN MAIN POSITION

      U     "Start_CoolingZone";
      U     "DB_GRP_71".VA21.SM.Close;
      U     "DB_GRP_71".FLA02.SM.Open;
      U(    ;
      O     "DB_GRP_71".FLA12_M1.SM.Open;
      O(    ;
      L     "DB_GRP_71".FLA12_M1.PV.Position;
      L     5.900000e+001;
      >=R   ;
      )     ;
      )     ;
      U(    ;
      O     "DB_GRP_71".FLA12_M2.SM.Open;
      O     "DB_PROG".OVEN.SM.AggregateEmptied;
      )     ;
      =     "CoolingZone_Set_MP";
NETWORK
TITLE =START FANS OF COOLING ZONE

      U     "Start_CoolingZone";
      U     "CoolingZone_Set_MP";
      UN    "DB_Gest_ES".FLAG._002;
      S     "StartFans_CoolZone";
      U(    ;
      U     "CoolZone_OFF";
      U(    ;
      O     "DB_GRP_71".FLA12_M1.SM.Close;
      O     ;
      UN    "DB_PROG".OVEN.SM.CoolingZoneON;
      UN    "Start_CoolingZone";
      )     ;
      O     "DB_MULFUNCTION".SM.CZ_MALFUNCTION_STOP_L2;
      O     "DB_Gest_ES".FLAG._002;
      )     ;
      UN    "Timer_AfterRun_Done";
      R     "StartFans_CoolZone";
      NOP   0;
NETWORK
TITLE =TIMER T2_0_1. PAUSE TO START SUPPLY AIR FAN =31FAN31_M1
//WHEN FLAPS ARE IN MAIN (START) POSITION, SET TIMER DELAY AND START AIR FANS
//=31FAN31, =31FAN03, =31FAN01
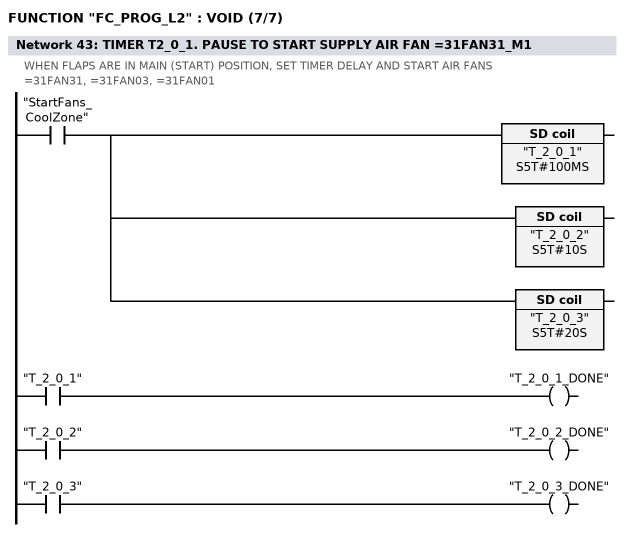
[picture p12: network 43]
      U     "StartFans_CoolZone";
      =     L      6.0;
      U     L      6.0;
      L     S5T#100MS;
      SE    "T_2_0_1";
      NOP   0;
      NOP   0;
      NOP   0;
      U     "T_2_0_1";
      =     "T_2_0_1_DONE";
      U     L      6.0;
      L     S5T#10S;
      SE    "T_2_0_2";
      NOP   0;
      NOP   0;
      NOP   0;
      U     "T_2_0_2";
      =     "T_2_0_2_DONE";
      U     L      6.0;
      L     S5T#20S;
      SE    "T_2_0_3";
      NOP   0;
      NOP   0;
      NOP   0;
      U     "T_2_0_3";
      =     "T_2_0_3_DONE";
NETWORK
TITLE =WHEN ALL FANS RUNNING AND PRESSURE SENSORS ARE OK
//WHEN TEMPERATURE IN ALL HEATING BOXES OK, FANS RUNNING AND PRESSURE SENSORS ARE
//OK - SET STATUS "RELEASE OF PRODUCTION OVEN" AND "RELEASE FOR CONVEYING"
      U(    ;
      U(    ;
      U     "DB_GRP_71".FAN01.SM.MotorOn;
      U     "DB_DIGIT".SM.G71_FAN01;
      O     "DB_Gest_ES".FLAG._014;
      O     "DB_Gest_ES".FLAG._002;
      )     ;
      U     "OvensTemperatureOK";
      L     S5T#1M;
      SA    "CONV_LINE2_PROD_REL_DEL";
      NOP   0;
      NOP   0;
      NOP   0;
      U     "CONV_LINE2_PROD_REL_DEL";
      )     ;
      U     "DB_MULFUNCTION".SM.RECIRC_FANS_OK_L2;
      U     "OvenFans_IsRun";
      U     "OvenFans_IsOn";
      U     "DB_PROG".OVEN.SM.ProductionON;
      UN    "DB_PROG".OVEN.SM.ProductionBreakON;
      UN    "DB_PROG".OVEN.SM.SwitchOffProduction;
      UN    "DB_PROG".OVEN.SM.EmergencyCoolingON;
      =     "DB_PROG".OVEN.SM.ProductionRelease;
NETWORK
TITLE =COOLING ZONE ON
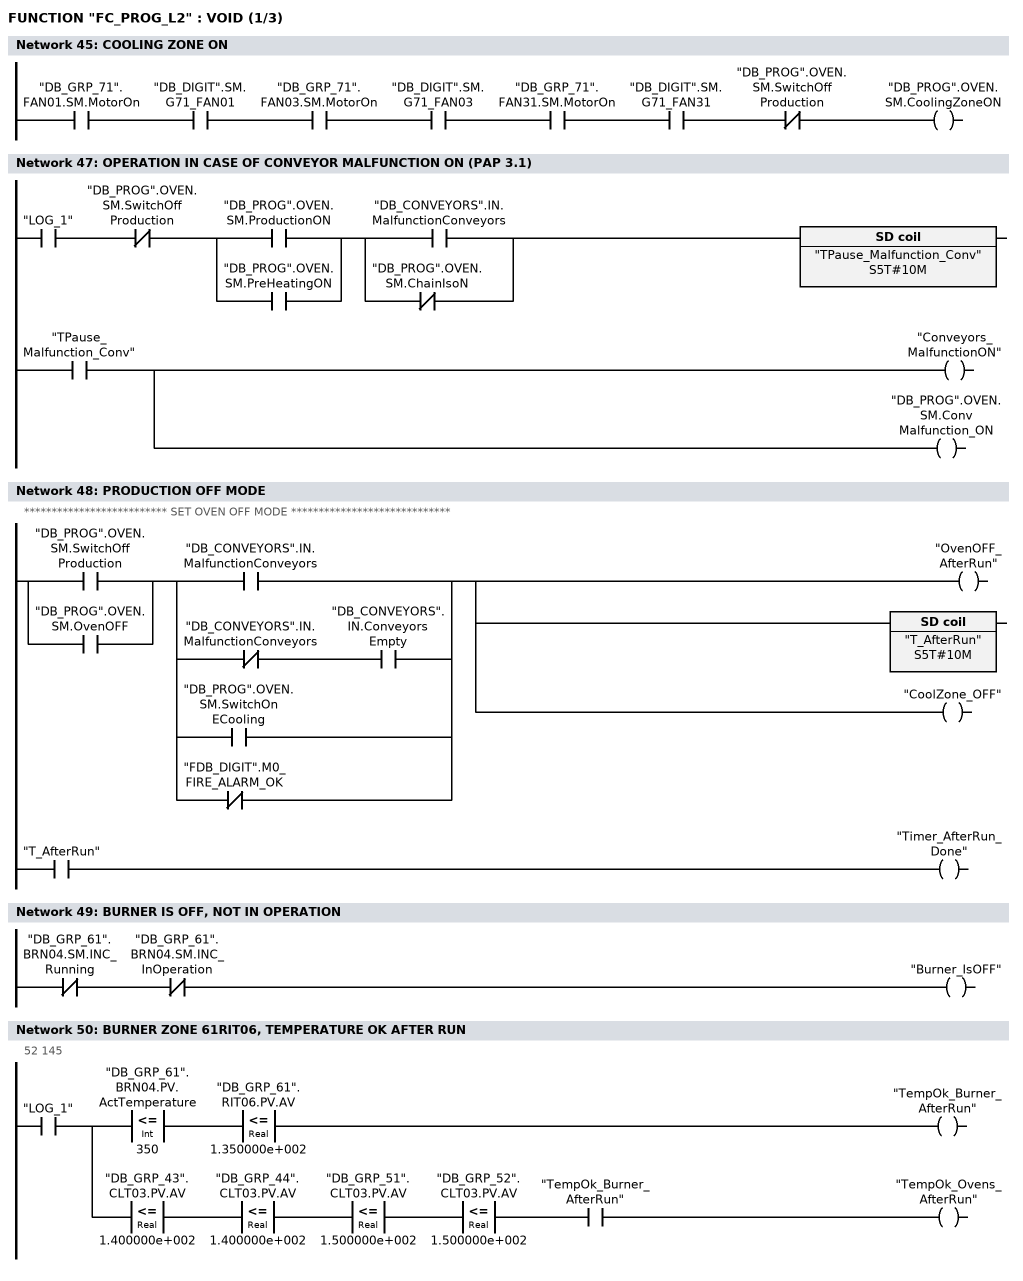
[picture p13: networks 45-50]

      U     "DB_GRP_71".FAN01.SM.MotorOn;
      U     "DB_DIGIT".SM.G71_FAN01;
      U     "DB_GRP_71".FAN03.SM.MotorOn;
      U     "DB_DIGIT".SM.G71_FAN03;
      U     "DB_GRP_71".FAN31.SM.MotorOn;
      U     "DB_DIGIT".SM.G71_FAN31;
      UN    "DB_PROG".OVEN.SM.SwitchOffProduction;
      =     "DB_PROG".OVEN.SM.CoolingZoneON;
NETWORK
TITLE =PRODUCTION BREAK MODE
//
//********************** SET OVEN PRODUCTION BREAK MODE ************************
//
NETWORK
TITLE =OPERATION IN CASE OF CONVEYOR MALFUNCTION ON (PAP 3.1)

      U     "LOG_1";
      UN    "DB_PROG".OVEN.SM.SwitchOffProduction;
      U(    ;
      O     "DB_PROG".OVEN.SM.ProductionON;
      O     "DB_PROG".OVEN.SM.PreHeatingON;
      )     ;
      U(    ;
      O     "DB_CONVEYORS".IN.MalfunctionConveyors;
      ON    "DB_PROG".OVEN.SM.ChainIsoN;
      )     ;
      L     S5T#10M;
      SE    "TPause_Malfunction_Conv";
      NOP   0;
      NOP   0;
      NOP   0;
      U     "TPause_Malfunction_Conv";
      =     "Conveyors_MalfunctionON";
      =     "DB_PROG".OVEN.SM.ConvMalfunction_ON;
NETWORK
TITLE =PRODUCTION OFF MODE
//
//************************** SET OVEN OFF MODE *****************************
//
//
      U(    ;
      O     "DB_PROG".OVEN.SM.SwitchOffProduction;
      O     "DB_PROG".OVEN.SM.OvenOFF;
      )     ;
      U(    ;
      O     "DB_CONVEYORS".IN.MalfunctionConveyors;
      O     ;
      UN    "DB_CONVEYORS".IN.MalfunctionConveyors;
      U     "DB_CONVEYORS".IN.ConveyorsEmpty;
      O     "DB_PROG".OVEN.SM.SwitchOnECooling;
      ON    "FDB_DIGIT".M0_FIRE_ALARM_OK;
      )     ;
      =     L      6.0;
      U     L      6.0;
      BLD   102;
      =     "OvenOFF_AfterRun";
      U     L      6.0;
      L     S5T#10M;
      SE    "T_AfterRun";
      NOP   0;
      NOP   0;
      NOP   0;
      U     "T_AfterRun";
      =     "Timer_AfterRun_Done";
      U     L      6.0;
      BLD   102;
      =     "CoolZone_OFF";
NETWORK
TITLE =BURNER IS OFF, NOT IN OPERATION

      UN    "DB_GRP_61".BRN04.SM.INC_Running;
      UN    "DB_GRP_61".BRN04.SM.INC_InOperation;
      =     "Burner_IsOFF";
NETWORK
TITLE =BURNER ZONE 61RIT06, TEMPERATURE OK AFTER RUN
//52 145
      U     "LOG_1";
      =     L      6.0;
      U     L      6.0;
      U(    ;
      L     "DB_GRP_61".BRN04.PV.ActTemperature;
      L     350;
      <=I   ;
      )     ;
      U(    ;
      L     "DB_GRP_61".RIT06.PV.AV;
      L     1.350000e+002;
      <=R   ;
      )     ;
      =     "TempOk_Burner_AfterRun";
      U     L      6.0;
      U(    ;
      L     "DB_GRP_43".CLT03.PV.AV;
      L     1.400000e+002;
      <=R   ;
      )     ;
      U(    ;
      L     "DB_GRP_44".CLT03.PV.AV;
      L     1.400000e+002;
      <=R   ;
      )     ;
      U(    ;
      L     "DB_GRP_51".CLT03.PV.AV;
      L     1.500000e+002;
      <=R   ;
      )     ;
      U(    ;
      L     "DB_GRP_52".CLT03.PV.AV;
      L     1.500000e+002;
      <=R   ;
      )     ;
      U     "TempOk_Burner_AfterRun";
      =     "TempOk_Ovens_AfterRun";
NETWORK
TITLE =OFF EXHAUST AIR FAN =60FAN01 AND FRESH AIR HEAT EXCHANGER FAN =1
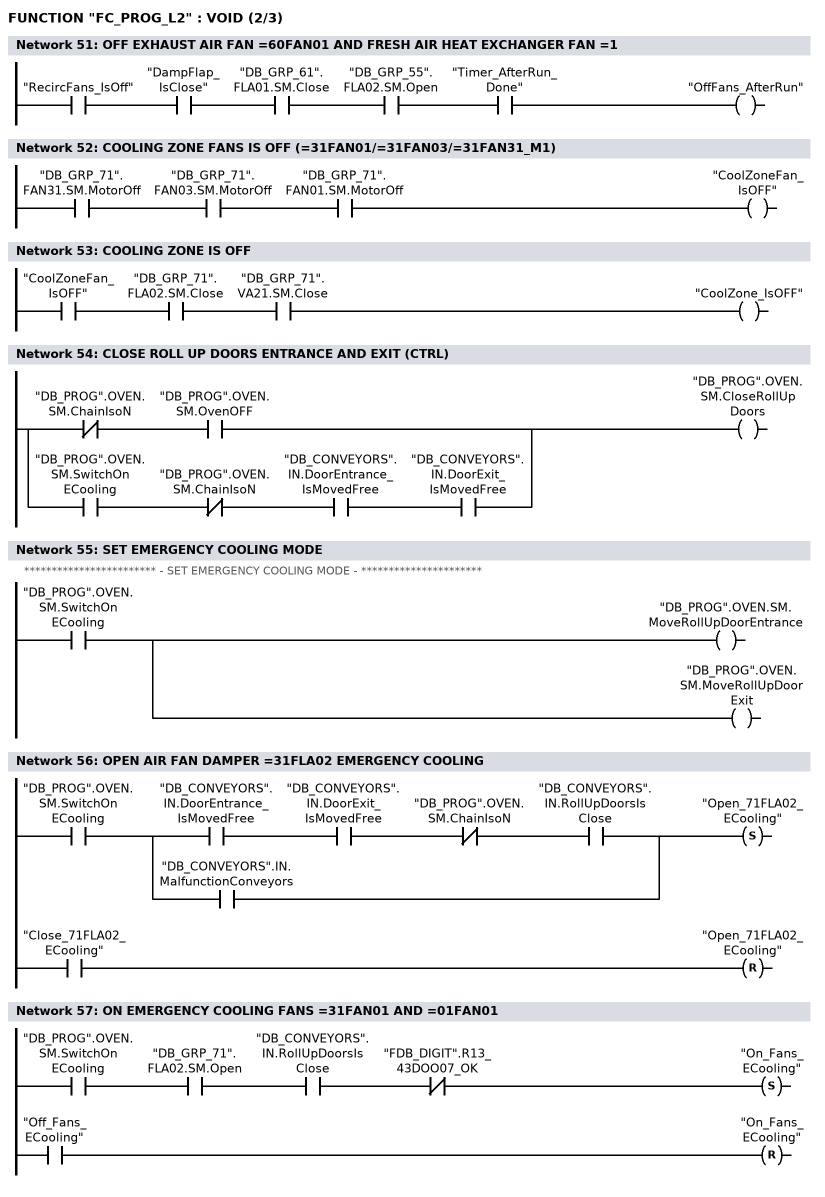
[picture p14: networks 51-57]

      U     "RecircFans_IsOff";
      U     "DampFlap_IsClose";
      U     "DB_GRP_61".FLA01.SM.Close;
      U     "DB_GRP_55".FLA02.SM.Open;
      U     "Timer_AfterRun_Done";
      =     "OffFans_AfterRun";
NETWORK
TITLE =COOLING ZONE FANS IS OFF (=31FAN01/=31FAN03/=31FAN31_M1)

      U     "DB_GRP_71".FAN31.SM.MotorOff;
      U     "DB_GRP_71".FAN03.SM.MotorOff;
      U     "DB_GRP_71".FAN01.SM.MotorOff;
      =     "CoolZoneFan_IsOFF";
NETWORK
TITLE =COOLING ZONE IS OFF

      U     "CoolZoneFan_IsOFF";
      U     "DB_GRP_71".FLA02.SM.Close;
      U     "DB_GRP_71".VA21.SM.Close;
      =     "CoolZone_IsOFF";
NETWORK
TITLE =CLOSE ROLL UP DOORS ENTRANCE AND EXIT (CTRL)

      UN    "DB_PROG".OVEN.SM.ChainIsoN;
      U     "DB_PROG".OVEN.SM.OvenOFF;
      O     ;
      U     "DB_PROG".OVEN.SM.SwitchOnECooling;
      UN    "DB_PROG".OVEN.SM.ChainIsoN;
      U     "DB_CONVEYORS".IN.DoorEntrance_IsMovedFree;
      U     "DB_CONVEYORS".IN.DoorExit_IsMovedFree;
      =     "DB_PROG".OVEN.SM.CloseRollUpDoors;
NETWORK
TITLE =SET EMERGENCY COOLING MODE
//
//************************ - SET EMERGENCY COOLING MODE - **********************
//
      U     "DB_PROG".OVEN.SM.SwitchOnECooling;
      =     "DB_PROG".OVEN.SM.MoveRollUpDoorEntrance;
      =     "DB_PROG".OVEN.SM.MoveRollUpDoorExit;
NETWORK
TITLE =OPEN AIR FAN DAMPER =31FLA02 EMERGENCY COOLING

      U     "DB_PROG".OVEN.SM.SwitchOnECooling;
      U(    ;
      U     "DB_CONVEYORS".IN.DoorEntrance_IsMovedFree;
      U     "DB_CONVEYORS".IN.DoorExit_IsMovedFree;
      UN    "DB_PROG".OVEN.SM.ChainIsoN;
      U     "DB_CONVEYORS".IN.RollUpDoorsIsClose;
      O     "DB_CONVEYORS".IN.MalfunctionConveyors;
      )     ;
      S     "Open_71FLA02_ECooling";
      U     "Close_71FLA02_ECooling";
      R     "Open_71FLA02_ECooling";
      NOP   0;
NETWORK
TITLE =ON EMERGENCY COOLING FANS =31FAN01 AND =01FAN01

      U     "DB_PROG".OVEN.SM.SwitchOnECooling;
      U     "DB_GRP_71".FLA02.SM.Open;
      U     "DB_CONVEYORS".IN.RollUpDoorsIsClose;
      UN    "FDB_DIGIT".R13_43DOO07_OK;
      S     "On_Fans_ECooling";
      U     "Off_Fans_ECooling";
      R     "On_Fans_ECooling";
      NOP   0;
NETWORK
TITLE =SET EMERGENCY COOLING TIME 180 MIN
//SET TIMER T_7_1_1
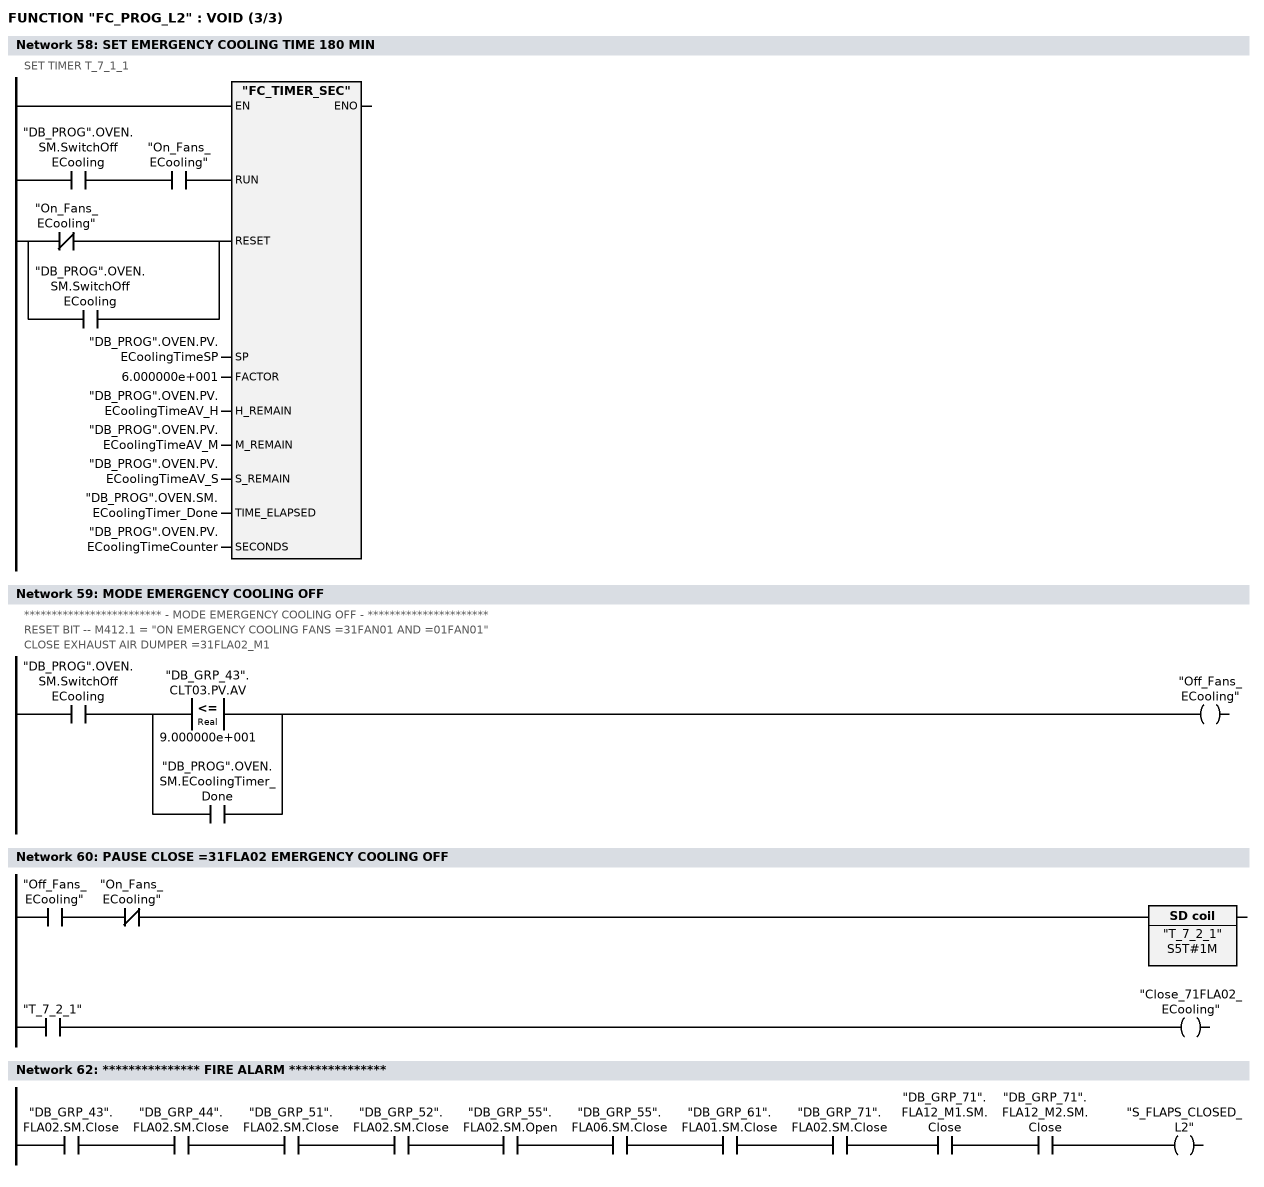
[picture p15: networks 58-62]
      U     "DB_PROG".OVEN.SM.SwitchOffECooling;
      U     "On_Fans_ECooling";
      =     L      6.0;
      BLD   103;
      U(    ;
      ON    "On_Fans_ECooling";
      O     "DB_PROG".OVEN.SM.SwitchOffECooling;
      )     ;
      =     L      6.1;
      BLD   103;
      CALL "FC_TIMER_SEC" (
           RUN                      := L      6.0,
           RESET                    := L      6.1,
           SP                       := "DB_PROG".OVEN.PV.ECoolingTimeSP,
           FACTOR                   := 6.000000e+001,
           H_REMAIN                 := "DB_PROG".OVEN.PV.ECoolingTimeAV_H,
           M_REMAIN                 := "DB_PROG".OVEN.PV.ECoolingTimeAV_M,
           S_REMAIN                 := "DB_PROG".OVEN.PV.ECoolingTimeAV_S,
           TIME_ELAPSED             := "DB_PROG".OVEN.SM.ECoolingTimer_Done,
           SECONDS                  := "DB_PROG".OVEN.PV.ECoolingTimeCounter);
      NOP   0;
NETWORK
TITLE =MODE EMERGENCY COOLING OFF
//
//************************* - MODE EMERGENCY COOLING OFF - **********************
//
//RESET BIT -- M412.1 = "ON EMERGENCY COOLING FANS =31FAN01 AND =01FAN01"
//CLOSE EXHAUST AIR DUMPER =31FLA02_M1
//
      U     "DB_PROG".OVEN.SM.SwitchOffECooling;
      U(    ;
      O(    ;
      L     "DB_GRP_43".CLT03.PV.AV;
      L     9.000000e+001;
      <=R   ;
      )     ;
      O     "DB_PROG".OVEN.SM.ECoolingTimer_Done;
      )     ;
      =     "Off_Fans_ECooling";
NETWORK
TITLE =PAUSE CLOSE =31FLA02 EMERGENCY COOLING OFF

      U     "Off_Fans_ECooling";
      UN    "On_Fans_ECooling";
      L     S5T#1M;
      SE    "T_7_2_1";
      NOP   0;
      NOP   0;
      NOP   0;
      U     "T_7_2_1";
      =     "Close_71FLA02_ECooling";
NETWORK
TITLE =********** END CYCLE OF OVEN *************

NETWORK
TITLE =*************** FIRE ALARM ***************

      U     "DB_GRP_43".FLA02.SM.Close;
      U     "DB_GRP_44".FLA02.SM.Close;
      U     "DB_GRP_51".FLA02.SM.Close;
      U     "DB_GRP_52".FLA02.SM.Close;
      U     "DB_GRP_55".FLA02.SM.Open;
      U     "DB_GRP_55".FLA06.SM.Close;
      U     "DB_GRP_61".FLA01.SM.Close;
      U     "DB_GRP_71".FLA02.SM.Close;
      U     "DB_GRP_71".FLA12_M1.SM.Close;
      U     "DB_GRP_71".FLA12_M2.SM.Close;
      =     "S_FLAPS_CLOSED_L2";
NETWORK
TITLE =END

END_FUNCTION

